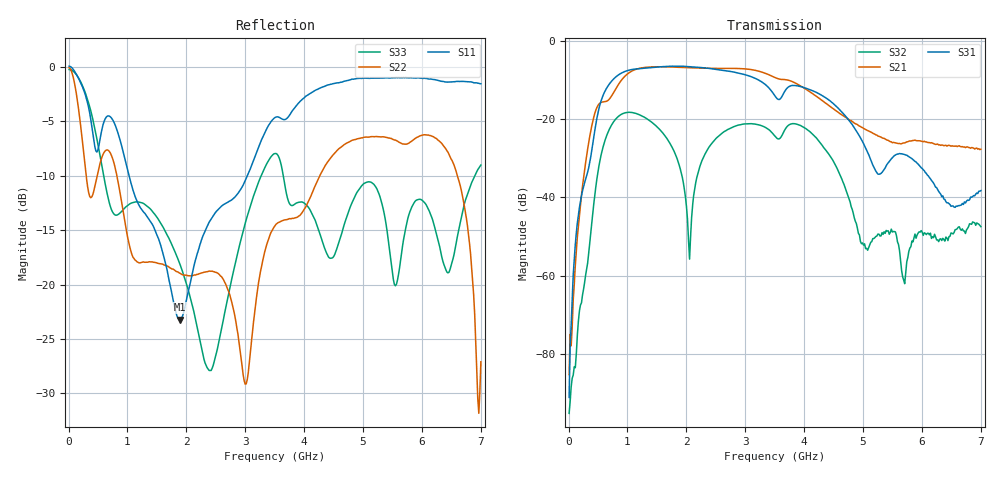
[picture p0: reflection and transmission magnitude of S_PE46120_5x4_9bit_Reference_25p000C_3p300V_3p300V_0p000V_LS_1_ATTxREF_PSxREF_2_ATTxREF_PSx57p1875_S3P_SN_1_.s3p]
! Device ID: PE46120_5x4_9bit_Reference
! Device ID: PE46120_5x4_9bit_Reference
! File Path: z:\PE46120_5x4_9bit_Reference\MPAC_Yi\new_12port\25p000C\3p300\LS_1_ATTxREF_PSxREF_2_ATTxREF_PSx57p1875\PE46120_5x4_9bit_Reference_25p000C_3p300V_3p300V_0p000V_LS_1_ATTxREF_PSxREF_2_ATTxREF_PSx57p1875_S3P_SN_1_.s3p
! Serial: 1
! Lot:
! Temp: 25.000C
! VDD: 3.300
! VSS: 0.000
! Control_Hi: 3.300
! Control_Lo: 0.000
! Logic State: LS_1_ATTxREF_PSxREF_2_ATTxREF_PSx57p1875
! Port 1: RFin
! Port 2: RFout1
! Port 3: RFout2
! ThroughPath:1-3
! IDD: -0.000547526
! ISS: 0
! Comment:
#  Hz  S  RI  R  50
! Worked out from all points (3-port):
!   401 points, 10 MHz to 7 GHz, reference 50 ohm
!   strongest paths, dB at 10 MHz, 1.758 GHz, 3.505 GHz, 5.253 GHz, 7 GHz:
!     S31: -91.2, -6.5, -14.1, -34.1, -38.3
!     S21: -85.3, -6.7, -9.4, -24.3, -27.7
!     S32: -95.2, -27.2, -24.3, -49.4, -47.5
!   lowest |S11| = -23.2 dB at 1.897 GHz (marker M1), VSWR 1.15, Z = 57.4 + j0.704 ohm
!   |S11| at or under -10 dB: 1.028 GHz to 3.035 GHz (2.007 GHz wide, 98.8 % of centre)
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1e7  1.001 -0.1149  0.000148 8.92e-05  4.83e-05 0.000107
     5.4e-05 6.95e-06  0.9871 -0.0966  9.43e-05 6.48e-05
     -2.52e-05 1.14e-05  1.56e-05 -7.43e-06  0.9709 -0.0481
2.37175e8  -0.4713 -0.6571  -0.0127 -0.00491  -0.0109 0.00475
           -0.013 -0.00492  -0.2852 -0.3502  -0.000395 0.000424
           -0.0111 0.00477  -0.000339 0.000449  0.3687 -0.7313
4.6435e8  -0.4046 -0.0705  -0.0562 0.1161  -0.071 0.0484
          -0.0567 0.1178  0.1376 0.264  0.00349 -0.0131
          -0.0717 0.0491  0.00356 -0.0133  -0.3171 -0.377
9.71125e8  -0.217 0.2927  0.3465 -0.0876  0.3754 -0.1523
           0.3507 -0.0891  -0.0495 -0.1769  0.1169 -0.025
           0.3799 -0.1546  0.1181 -0.0256  0.2055 0.0968
1.8973e9  0.0688 0.00611  -0.4202 0.1706  -0.4448 0.1481
          -0.4249 0.1731  -0.1069 0.0353  0.0168 0.0154
          -0.45 0.1505  0.017 0.0155  -0.0609 -0.1066
2.054575e9  0.0637 -0.0748  -0.3023 0.3312  -0.3291 0.3269
            -0.3054 0.3357  -0.0705 0.0839  -0.000517 0.00139
            -0.3323 0.3312  -0.000153 0.00161  -0.0632 -0.0637
2.49145e9  -0.0606 -0.205  0.1928 0.3953  0.1856 0.387
           0.1959 0.3996  0.0847 0.0761  0.0169 0.0516
           0.1886 0.3917  0.0172 0.0524  -0.0289 -0.0362
3.505e9  -0.4612 -0.3601  -0.0825 -0.325  -0.0153 -0.1948
         -0.0841 -0.3291  0.0657 0.1742  -0.0591 0.0104
         -0.0155 -0.197  -0.0597 0.0109  0.1519 0.3698
5.689375e9  -0.6552 0.6059  0.0482 0.00612  0.034 0.00833
            0.0492 0.00598  0.3609 0.2555  6.54e-05 0.000127
            0.0344 0.00869  0.000638 0.0006  0.1026 0.1256
7e9  -0.0828 0.8323  -0.0232 -0.0331  0.0111 -0.00502
     -0.0231 -0.0342  -0.0331 0.0292  0.00389 0.00317
     0.0111 -0.00497  0.00309 0.00287  0.11 0.3365
